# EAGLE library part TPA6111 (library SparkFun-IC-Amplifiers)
TPA6111A2 Basic 150mW stereo headphone amplifier. SparkFun Products SparkFun FM Tuner Evaluation Board - Si4703 (WRL-12938)
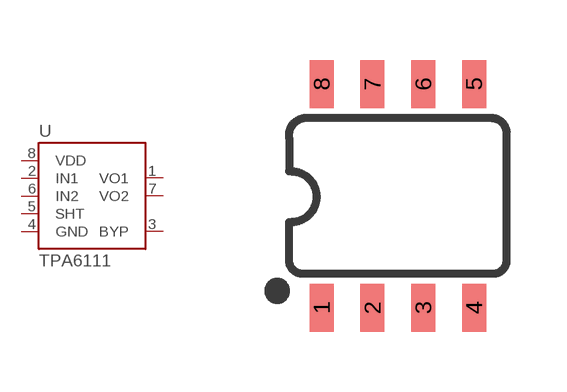
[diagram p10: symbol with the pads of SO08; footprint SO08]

Designator prefix U

## TPA6111SMD-T (PROD_ID: IC-10149; VALUE: TPA6111A2DR)  [SO08]
1  VO1
2  IN1
3  BYP
4  GND
5  SHT
6  IN2
7  VO2
8  VDD

## Footprint SO08 (pad centres in mm)
SOIC, 0.15 inch width
smd 0.6 x 1.2: 1 -1.905,-2.8; 2 -0.635,-2.8; 3 0.635,-2.8; 4 1.905,-2.8; 5 1.905,2.8; 6 0.635,2.8; 7 -0.635,2.8; 8 -1.905,2.8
